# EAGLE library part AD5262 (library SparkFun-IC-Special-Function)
Digital Potentiometer IC Datasheet SparkFun Products SparkFun Touch Potentiometer (PRT-13144)
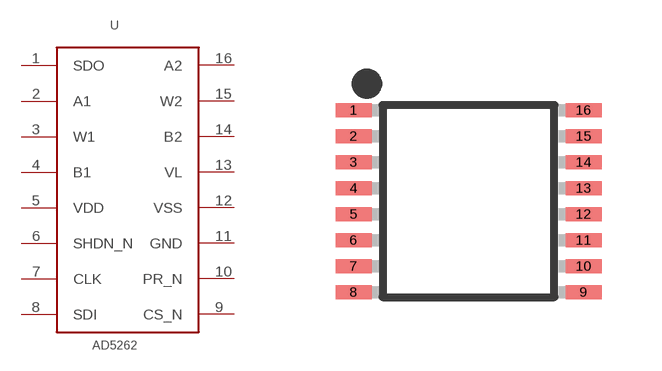
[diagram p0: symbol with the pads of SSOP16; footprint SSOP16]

Designator prefix -

## AD5262 (PROD_ID: IC-12358; VALUE: AD5262BRU)  [SSOP16]
1  SDO  out
2  A1  pas
3  W1  pas
4  B1  pas
5  VDD  pwr
6  SHDN_N  in
7  CLK  in
8  SDI  in
9  CS_N  in
10  PR_N  in
11  GND  pwr
12  VSS  pwr
13  VL  pwr
14  B2  pas
15  W2  pas
16  A2  pas

## Footprint SSOP16 (pad centres in mm)
smd 0.9 x 0.35: 1 -2.875,2.275; 2 -2.875,1.625; 3 -2.875,0.975; 4 -2.875,0.325; 5 -2.875,-0.325; 6 -2.875,-0.975; 7 -2.875,-1.625; 8 -2.875,-2.275; 9 2.875,-2.275; 10 2.875,-1.625; 11 2.875,-0.975; 12 2.875,-0.325; 13 2.875,0.325; 14 2.875,0.975; 15 2.875,1.625; 16 2.875,2.275

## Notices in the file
Licensing: Creative Commons ShareAlike 4.0 International - https://creativecommons.org/licenses/by-sa/4.0
